(* Logix 5000 AddOnInstructionDefinition export EH_Liquitrend_QMW43_IOL; software revision 38.00 *)

TYPE EH_CommAOI_Data :
STRUCT
   Device_Comm_Error : BOOL;
   CommSuccess : BOOL;
   CommFailed : BOOL;
   CommTimeOut : BOOL;
   StateDone : BOOL;
   NewState : BOOL;
   OldState : SINT;
   PortSize : SINT;
   DevicePort : SINT;
   MaxState : SINT;
   State : SINT;
   VendorID : INT;
   DeviceID : DINT;
   CyclicData : INT[16];
   AcyclicData : DINT[8];
   ReplayIndex : INT;
   AOI_Diagnostic : DINT;
   ConnectionStatus : DINT;
   OutputData : INT[16];
END_STRUCT
END_TYPE

ADD_ON_INSTRUCTION EH_Liquitrend_QMW43_IOL   (* revision 1.0, vendor Endress+Hauser *)
// Liquitrend QMW43  Rev 1 IO-Link
VAR_IN_OUT
   DataToSend : INT[10]; {required}
   CommAOIBusy : DINT; {required}
   ActiveComPort : DINT; {required}
   DeviceAOISendRequest : DINT; {required}
   CommError : INT; {required}
   DeviceData : EH_CommAOI_Data; {required}
END_VAR
VAR_INPUT
   iExecuteRisingEdge : BOOL; {visible}
   iSetSimulation_Conductivity_Active : BOOL; {visible}
   iSetSimulation_Conductivity_Value : DINT; {visible}
   iSetSimulation_BuildUp_Active : BOOL; {visible}
   iSetSimulation_BuildUp_Value : INT; {visible}
END_VAR
VAR_OUTPUT
   qVendor_ID : DINT; {access Read Only, visible}
   qDevice_ID : DINT; {access Read Only, visible}
   qConductivity : REAL; {visible}
   qSimulationConductivityActive : BOOL; {visible}
   qBuildUp : REAL; {visible}
   qSimulationBuildUpActive : BOOL; {access Read Only, visible}
   qAOI_Diagnostic : DINT; {access Read Only, visible}
END_VAR
VAR_IN_OUT
   qActual_Diagnostics_String : STRING; {required}
END_VAR
VAR_OUTPUT
   qActual_Diagnostics_Code : DINT; {access Read Only, visible}
END_VAR
VAR_IN_OUT
   qLast_Diagnostics_String : STRING; {required}
END_VAR
VAR_OUTPUT
   qLast_Diagnostics_Code : DINT; {access Read Only, visible}
   qCommunicationBusy : DINT; {visible}
   qCommError : INT; {access Read Only, visible}
   qDeviceConnectionError : BOOL; {access Read Only, visible}
END_VAR
VAR
   Calc_DID : DINT; {access None}
   Calc_VID : DINT; {access None}
   Calc_Data : DINT; {access None}
   Conductivity_DINT : DINT; {access None}
   Calc_Conductivity : DINT; {access None}
   Calc_CondenStatus : DINT; {access None}
   CMD_Index : INT; {access None}
   CMD_Subindex : INT; {access None}
   CMD_ByteLength : INT; {access None}
   Calc_Connection_Status : DINT; {access None}
   Trigger : BOOL; {access None}
   CMD_Rd : BOOL; {access None}
   CMD_Wr : BOOL; {access None}
   Calc_Out : DINT; {access None}
   UnitSelection : REAL; {access None}
   InputByteLength : DINT;
   LocalChannel : BOOL; {access None}
   StateMin : DINT; {access None}
   UseDeviceUnit : BOOL; {access None}
   ActiveAOI : BOOL; {access None}
   firstTimeDone : BOOL; {access None}
   AOI_Prio : BOOL; {access None}
   BuidlUp_DINT : DINT;
   SimulationDINT : DINT; {access None}
   DeviceID1 : DINT; {access None}
   FALSE : BOOL; {access None}
   TRUE : BOOL := 1; {access None}
END_VAR

ROUTINE Logic   (* structured text *)
// PMP23 Communication via AL1323
   // ©Copyright (2024) All Rights Reserved
   // =======================================================================
   // Name:                EH_Liquitrend_QMW43_IOL
   // Version:             1.0
   // Datum:               11.2025
   // Library:             01.01.00
   // Engineering:         Studio5000 V38.00.00
   // Author:              EH
   // =======================================================================
   
   
   qAOI_Diagnostic := DeviceData.AOI_Diagnostic;
   qCommunicationBusy := CommAOIBusy;
   DeviceID1 := 1536;
   StateMin := 0;
   DeviceData.MaxState := 9;
   
   if DeviceData.DevicePort = 0 or DeviceData.DeviceID <> DeviceID1 or DeviceData.ConnectionStatus <> 1 then
   
   	qVendor_ID	:= 0;
   	qDevice_ID	:= 0;
   	qConductivity	:= 0;
   	qBuildUp	:=0;
   	qSimulationBuildUpActive	:= 0;
   	qSimulationConductivityActive	:= 0;
   	qActual_Diagnostics_Code	:= 0;
   	qLast_Diagnostics_Code	:= 0;
   	qLast_Diagnostics_String	:= '';
   
   	if DeviceData.DevicePort = 0 then
   
   		qActual_Diagnostics_String	:= 'Device Port is Zero';
   		DeviceData.AOI_Diagnostic.1 := TRUE;
   
   	elsif DeviceData.ConnectionStatus <> 1 then
   
   		qActual_Diagnostics_String	:= 'No Device connected';
   		qDeviceConnectionError := TRUE;
   
   	elsif DeviceData.DeviceID <> DeviceID1 then
   
   		qActual_Diagnostics_String	:= 'Wrong DeviceID';
   		DeviceData.AOI_Diagnostic.2 := TRUE;
   		qVendor_ID := DeviceData.VendorID;
   		qDevice_ID := DeviceData.DeviceID;
   
   	end_if;
   
   else
   
   	if qActual_Diagnostics_Code = 0 then
   
   		qActual_Diagnostics_String	:= '--------';
   
   	end_if;
   
   	if qLast_Diagnostics_Code = 0 then
   
   		qLast_Diagnostics_String	:= '--------';
   
   	end_if;
   
   	DeviceData.AOI_Diagnostic.1 := FALSE;
   	qDeviceConnectionError := FALSE;
   	DeviceData.AOI_Diagnostic.2  := FALSE;
   
   end_if;
   
   if NOT DeviceData.AOI_Diagnostic.0
   	and not qDeviceConnectionError
   	and not DeviceData.AOI_Diagnostic.2
   	and DeviceData.DevicePort > 0 or ActiveAOI and qDeviceConnectionError then
   
   	//*********************************
   	//Vendor ID
   	//*********************************
   
   	qVendor_ID := DeviceData.VendorID;
   
   	//*********************************
   	//Device ID
   	//*********************************
   
   	qDevice_ID := DeviceData.DeviceID;
   
   	//*********************************
   	//Process Data Conductivity
   	//*********************************
   
   		Calc_Conductivity := 0+((DeviceData.DevicePort-1)*InputByteLength);	// Value  95 + Protnumber x Datalength 32 Byte
   
   		Conductivity_DINT := DeviceData.CyclicData[Calc_Conductivity+1];
   		Conductivity_DINT.16 := DeviceData.CyclicData[Calc_Conductivity].0;
   		Conductivity_DINT.17 := DeviceData.CyclicData[Calc_Conductivity].1;
   		Conductivity_DINT.18 := DeviceData.CyclicData[Calc_Conductivity].2;
   		Conductivity_DINT.19 := DeviceData.CyclicData[Calc_Conductivity].3;
   		Conductivity_DINT.20 := DeviceData.CyclicData[Calc_Conductivity].4;
   		Conductivity_DINT.21 := DeviceData.CyclicData[Calc_Conductivity].5;
   		Conductivity_DINT.22 := DeviceData.CyclicData[Calc_Conductivity].6;
   		Conductivity_DINT.23 := DeviceData.CyclicData[Calc_Conductivity].7;
   		Conductivity_DINT.24 := DeviceData.CyclicData[Calc_Conductivity].7;
   		Conductivity_DINT.25 := DeviceData.CyclicData[Calc_Conductivity].7;
   		Conductivity_DINT.26 := DeviceData.CyclicData[Calc_Conductivity].7;
   		Conductivity_DINT.27 := DeviceData.CyclicData[Calc_Conductivity].7;
   		Conductivity_DINT.28 := DeviceData.CyclicData[Calc_Conductivity].7;
   		Conductivity_DINT.29 := DeviceData.CyclicData[Calc_Conductivity].7;
   		Conductivity_DINT.30 := DeviceData.CyclicData[Calc_Conductivity].7;
   		Conductivity_DINT.31 := DeviceData.CyclicData[Calc_Conductivity].7;
   		/*
   		Conductivity_DINT.0 := DeviceData.CyclicData[Calc_Conductivity+1].8;
   		Conductivity_DINT.1 := DeviceData.CyclicData[Calc_Conductivity+1].9;
   		Conductivity_DINT.2 := DeviceData.CyclicData[Calc_Conductivity+1].10;
   		Conductivity_DINT.3 := DeviceData.CyclicData[Calc_Conductivity+1].11;
   		Conductivity_DINT.4 := DeviceData.CyclicData[Calc_Conductivity+1].12;
   		Conductivity_DINT.5 := DeviceData.CyclicData[Calc_Conductivity+1].13;
   		Conductivity_DINT.6 := DeviceData.CyclicData[Calc_Conductivity+1].14;
   		Conductivity_DINT.7 := DeviceData.CyclicData[Calc_Conductivity+1].15;
   		Conductivity_DINT.8 := DeviceData.CyclicData[Calc_Conductivity+1].0;
   		Conductivity_DINT.9 := DeviceData.CyclicData[Calc_Conductivity+1].1;
   		Conductivity_DINT.10 := DeviceData.CyclicData[Calc_Conductivity+1].2;
   		Conductivity_DINT.11 := DeviceData.CyclicData[Calc_Conductivity+1].3;
   		Conductivity_DINT.12 := DeviceData.CyclicData[Calc_Conductivity+1].4;
   		Conductivity_DINT.13 := DeviceData.CyclicData[Calc_Conductivity+1].5;
   		Conductivity_DINT.14 := DeviceData.CyclicData[Calc_Conductivity+1].6;
   		Conductivity_DINT.15 := DeviceData.CyclicData[Calc_Conductivity+1].7;
   		Conductivity_DINT.16 := DeviceData.CyclicData[Calc_Conductivity].0;
   		Conductivity_DINT.17 := DeviceData.CyclicData[Calc_Conductivity].1;
   		Conductivity_DINT.18 := DeviceData.CyclicData[Calc_Conductivity].2;
   		Conductivity_DINT.19 := DeviceData.CyclicData[Calc_Conductivity].3;
   		Conductivity_DINT.20 := DeviceData.CyclicData[Calc_Conductivity].4;
   		Conductivity_DINT.21 := DeviceData.CyclicData[Calc_Conductivity].5;
   		Conductivity_DINT.22 := DeviceData.CyclicData[Calc_Conductivity].6;
   		Conductivity_DINT.23 := DeviceData.CyclicData[Calc_Conductivity].7;
   		Conductivity_DINT.24 := DeviceData.CyclicData[Calc_Conductivity].7;
   		Conductivity_DINT.25 := DeviceData.CyclicData[Calc_Conductivity].7;
   		Conductivity_DINT.26 := DeviceData.CyclicData[Calc_Conductivity].7;
   		Conductivity_DINT.27 := DeviceData.CyclicData[Calc_Conductivity].7;
   		Conductivity_DINT.28 := DeviceData.CyclicData[Calc_Conductivity].7;
   		Conductivity_DINT.29 := DeviceData.CyclicData[Calc_Conductivity].7;
   		Conductivity_DINT.30 := DeviceData.CyclicData[Calc_Conductivity].7;
   		Conductivity_DINT.31 := DeviceData.CyclicData[Calc_Conductivity].7;
   		*/
   
   		qConductivity := Conductivity_DINT;
   		qConductivity := qConductivity/10;
   
   	//*********************************
   	//Process Data BuildUp
   	//*********************************
   
   		BuidlUp_DINT.0 := DeviceData.CyclicData[Calc_Conductivity].8;
   		BuidlUp_DINT.1 := DeviceData.CyclicData[Calc_Conductivity].9;
   		BuidlUp_DINT.2 := DeviceData.CyclicData[Calc_Conductivity].10;
   		BuidlUp_DINT.3 := DeviceData.CyclicData[Calc_Conductivity].11;
   		BuidlUp_DINT.4 := DeviceData.CyclicData[Calc_Conductivity].12;
   		BuidlUp_DINT.5 := DeviceData.CyclicData[Calc_Conductivity].13;
   		BuidlUp_DINT.6 := DeviceData.CyclicData[Calc_Conductivity].14;
   		BuidlUp_DINT.7 := DeviceData.CyclicData[Calc_Conductivity].15;
   		BuidlUp_DINT.8 := DeviceData.CyclicData[Calc_Conductivity].15;
   		BuidlUp_DINT.9 := DeviceData.CyclicData[Calc_Conductivity].15;
   		BuidlUp_DINT.10 := DeviceData.CyclicData[Calc_Conductivity].15;
   		BuidlUp_DINT.11 := DeviceData.CyclicData[Calc_Conductivity].15;
   		BuidlUp_DINT.12 := DeviceData.CyclicData[Calc_Conductivity].15;
   		BuidlUp_DINT.13 := DeviceData.CyclicData[Calc_Conductivity].15;
   		BuidlUp_DINT.14 := DeviceData.CyclicData[Calc_Conductivity].15;
   		BuidlUp_DINT.15 := DeviceData.CyclicData[Calc_Conductivity].15;
   		BuidlUp_DINT.16 := DeviceData.CyclicData[Calc_Conductivity].15;
   		BuidlUp_DINT.17 := DeviceData.CyclicData[Calc_Conductivity].15;
   		BuidlUp_DINT.18 := DeviceData.CyclicData[Calc_Conductivity].15;
   		BuidlUp_DINT.19 := DeviceData.CyclicData[Calc_Conductivity].15;
   		BuidlUp_DINT.20 := DeviceData.CyclicData[Calc_Conductivity].15;
   		BuidlUp_DINT.21 := DeviceData.CyclicData[Calc_Conductivity].15;
   		BuidlUp_DINT.22 := DeviceData.CyclicData[Calc_Conductivity].15;
   		BuidlUp_DINT.23 := DeviceData.CyclicData[Calc_Conductivity].15;
   		BuidlUp_DINT.24 := DeviceData.CyclicData[Calc_Conductivity].15;
   		BuidlUp_DINT.25 := DeviceData.CyclicData[Calc_Conductivity].15;
   		BuidlUp_DINT.26 := DeviceData.CyclicData[Calc_Conductivity].15;
   		BuidlUp_DINT.27 := DeviceData.CyclicData[Calc_Conductivity].15;
   		BuidlUp_DINT.28 := DeviceData.CyclicData[Calc_Conductivity].15;
   		BuidlUp_DINT.29 := DeviceData.CyclicData[Calc_Conductivity].15;
   		BuidlUp_DINT.30 := DeviceData.CyclicData[Calc_Conductivity].15;
   		BuidlUp_DINT.31 := DeviceData.CyclicData[Calc_Conductivity].15;
   
   		qBuildUp := BuidlUp_DINT;
   		qBuildUp := qBuildUp/10;
   
   	//*********************************
   	// Checking for CommBlockBusy
   	//*********************************
   
   	if iExecuteRisingEdge and DeviceData.State = 0 then
   
   		DeviceAOISendRequest.[DeviceData.DevicePort] := 1;
   
   	end_if;
   
   	if ActiveComPort = DeviceData.DevicePort then
   
   		AOI_Prio :=1;
   	else
   
   		AOI_Prio := 0;
   	end_if;
   
   	if CommAOIBusy = 1 and iExecuteRisingEdge and DeviceData.State = 0 and AOI_Prio then
   
   		ActiveAOI := 1;
   
   	end_if;
   
   	qCommunicationBusy := CommAOIBusy;
   	qAOI_Diagnostic := DeviceData.AOI_Diagnostic;
   
   	if  ActiveAOI and qDeviceConnectionError then
   
   		DeviceData.State := DeviceData.MaxState;
   
   	end_if;
   
   	//*********************************
   	// State machine
   	//*********************************
   
   if ActiveAOI or DeviceData.State = DeviceData.MaxState then
   
   	case DeviceData.State of
   
   	    //*********************************
   	    0: // Idle
   	    //*********************************
   
   	    // Initializing
   	   		Trigger := 0;
   		    CMD_Index := 0;
   			CMD_Subindex := 0;
   	        CMD_Wr := 0;
   			CMD_Rd := 0;
   	        CMD_ByteLength := 0;
   
   			if DeviceData.DevicePort = ActiveComPort then // check if Device is Active to reset success
   					DeviceData.CommSuccess := 0;
   					DeviceData.CommTimeOut := 0;
   					DeviceData.NewState := 1;
   					DeviceData.StateDone := 0;
   			end_if;
   
   		    // Wait for trigger
   		    if iExecuteRisingEdge and ActiveComPort = DeviceData.DevicePort then
   
   				DeviceData.AOI_Diagnostic := 0;
   				DeviceData.State := DeviceData.State + 1;
   
   		    end_if;
   
   		//*********************************
   	    1: // Set Simulation Value Conductivity
   	    //*********************************
   
   	        CMD_Index := 86;
   	        CMD_Subindex := 0;
   	        CMD_Wr := 1;
   			CMD_Rd := 0;
   	        CMD_ByteLength := 4;
   			DataToSend[6]:= 0;
   			DataToSend[7]:= 0;
   
   			if iSetSimulation_Conductivity_Value <= 1100000 AND iSetSimulation_Conductivity_Value >= 0 then
   
   				COP(iSetSimulation_Conductivity_Value,SimulationDINT,1); // Copie the Bits from the Real in a DINT
   
   				DataToSend[6].0 :=  SimulationDINT.24;
   				DataToSend[6].1 :=  SimulationDINT.25;
   				DataToSend[6].2 :=  SimulationDINT.26;
   				DataToSend[6].3 :=  SimulationDINT.27;
   				DataToSend[6].4 :=  SimulationDINT.28;
   				DataToSend[6].5 :=  SimulationDINT.29;
   				DataToSend[6].6 :=  SimulationDINT.30;
   				DataToSend[6].7 :=  SimulationDINT.31;
   				DataToSend[6].8 :=  SimulationDINT.16;
   				DataToSend[6].9 :=  SimulationDINT.17;
   				DataToSend[6].10 := SimulationDINT.18;
   				DataToSend[6].11 := SimulationDINT.19;
   				DataToSend[6].12 := SimulationDINT.20;
   				DataToSend[6].13 := SimulationDINT.21;
   				DataToSend[6].14 := SimulationDINT.22;
   				DataToSend[6].15 := SimulationDINT.23;
   				DataToSend[7].0  := SimulationDINT.8;
   				DataToSend[7].1  := SimulationDINT.9;
   				DataToSend[7].2  := SimulationDINT.10;
   				DataToSend[7].3  := SimulationDINT.11;
   				DataToSend[7].4  := SimulationDINT.12;
   				DataToSend[7].5  := SimulationDINT.13;
   				DataToSend[7].6  := SimulationDINT.14;
   				DataToSend[7].7  := SimulationDINT.15;
   				DataToSend[7].8  := SimulationDINT.0;
   				DataToSend[7].9  := SimulationDINT.1;
   				DataToSend[7].10 := SimulationDINT.2;
   				DataToSend[7].11 := SimulationDINT.3;
   				DataToSend[7].12 := SimulationDINT.4;
   				DataToSend[7].13 := SimulationDINT.5;
   				DataToSend[7].14 := SimulationDINT.6;
   				DataToSend[7].15 := SimulationDINT.7;
   
   				Trigger := 1;
   
   				if DeviceData.NewState then
   
   					DeviceData.StateDone := 1;
   
   				end_if;
   
   				if  DeviceData.CommSuccess and DeviceData.ReplayIndex = CMD_Index then
   
   					Trigger := 0;
   					DeviceData.OldState := DeviceData.State;
   		    	    DeviceData.State := DeviceData.State + 1;
   					DeviceData.CommSuccess := 0;
   					DeviceData.AcyclicData[0] := 0;
   					DeviceData.NewState := 1;
   
   				 elsif DeviceData.CommTimeOut then
   
   					DeviceData.AOI_Diagnostic.[DeviceData.State+7] := 1;
   					DeviceData.OldState := DeviceData.State;
   		    	    DeviceData.State := DeviceData.State + 1;
   					DeviceData.CommTimeOut := 0;
   					DeviceData.AcyclicData[0] := 0;
   					DeviceData.NewState := 1;
   
   		    	end_if;
   
   			else
   
   				DeviceData.AOI_Diagnostic.[DeviceData.State+7] := 1;
   				DeviceData.OldState := DeviceData.State;
   		        DeviceData.State := DeviceData.State + 1;
   				DeviceData.CommTimeOut := 0;
   				DeviceData.AcyclicData[0] := 0;
   				DeviceData.NewState := 1;
   
   			end_if;
   
   		//*********************************
   		2: // Set Simulation Conductivity
   		//*********************************
   
   	        CMD_Index := 90;
   	        CMD_Subindex := 0;
   	        CMD_Wr := 1;
   			CMD_Rd := 0;
   	        CMD_ByteLength := 1;
   			DataToSend[6]:= 0;
   			DataToSend[7]:= 0;
   
   			DataToSend[6].0 := iSetSimulation_Conductivity_Active;
   			Trigger := 1;
   
   			if DeviceData.NewState then
   
   				DeviceData.StateDone := 1;
   
   			end_if;
   
   			if  DeviceData.CommSuccess and DeviceData.ReplayIndex = CMD_Index then
   
   					Trigger := 0;
   					DeviceData.OldState := DeviceData.State;
   			        DeviceData.State := DeviceData.State + 1;
   					DeviceData.CommSuccess := 0;
   					DeviceData.AcyclicData[0] := 0;
   					DeviceData.NewState := 1;
   
   			 elsif DeviceData.CommTimeOut then
   
   					DeviceData.AOI_Diagnostic.[DeviceData.State+7] := 1;
   					DeviceData.OldState := DeviceData.State;
   			        DeviceData.State := DeviceData.State + 1;
   					DeviceData.CommTimeOut := 0;
   					DeviceData.AcyclicData[0] := 0;
   					DeviceData.NewState := 1;
   
   			   end_if;
   
   		//*********************************
   	    3: // Set Simulation Value BuildUP
   	    //*********************************
   
   	        CMD_Index := 85;
   	        CMD_Subindex := 0;
   	        CMD_Wr := 1;
   			CMD_Rd := 0;
   	        CMD_ByteLength := 2;
   			DataToSend[6]:= 0;
   			DataToSend[7]:= 0;
   
   			if iSetSimulation_BuildUp_Value <= 100 or iSetSimulation_BuildUp_Value >= 0 then
   
   				COP(iSetSimulation_BuildUp_Value,SimulationDINT,1); // Copie the Bits from the Real in a DINT
   
   				DataToSend[6].0  := SimulationDINT.8;
   				DataToSend[6].1  := SimulationDINT.9;
   				DataToSend[6].2  := SimulationDINT.10;
   				DataToSend[6].3  := SimulationDINT.11;
   				DataToSend[6].4  := SimulationDINT.12;
   				DataToSend[6].5  := SimulationDINT.13;
   				DataToSend[6].6  := SimulationDINT.14;
   				DataToSend[6].7  := SimulationDINT.15;
   				DataToSend[6].8  := SimulationDINT.0;
   				DataToSend[6].9  := SimulationDINT.1;
   				DataToSend[6].10 := SimulationDINT.2;
   				DataToSend[6].11 := SimulationDINT.3;
   				DataToSend[6].12 := SimulationDINT.4;
   				DataToSend[6].13 := SimulationDINT.5;
   				DataToSend[6].14 := SimulationDINT.6;
   				DataToSend[6].15 := SimulationDINT.7;
   
   				Trigger := 1;
   
   				if DeviceData.NewState then
   
   					DeviceData.StateDone := 1;
   
   				end_if;
   
   				if  DeviceData.CommSuccess and DeviceData.ReplayIndex = CMD_Index then
   
   					Trigger := 0;
   					DeviceData.OldState := DeviceData.State;
   			        DeviceData.State := DeviceData.State + 1;
   					DeviceData.CommSuccess := 0;
   					DeviceData.AcyclicData[0] := 0;
   					DeviceData.NewState := 1;
   
   				 elsif DeviceData.CommTimeOut then
   
   					DeviceData.AOI_Diagnostic.[DeviceData.State+7] := 1;
   					DeviceData.OldState := DeviceData.State;
   			        DeviceData.State := DeviceData.State + 1;
   					DeviceData.CommTimeOut := 0;
   					DeviceData.AcyclicData[0] := 0;
   					DeviceData.NewState := 1;
   
   			    end_if;
   
   			else
   
   				DeviceData.AOI_Diagnostic.[DeviceData.State+7] := 1;
   				DeviceData.OldState := DeviceData.State;
   		        DeviceData.State := DeviceData.State + 1;
   				DeviceData.CommTimeOut := 0;
   				DeviceData.AcyclicData[0] := 0;
   				DeviceData.NewState := 1;
   
   			end_if;
   
   
   		//*********************************
   		4: // Set Simulation BuildUP
   		//*********************************
   
   	        CMD_Index := 66;
   	        CMD_Subindex := 0;
   	        CMD_Wr := 1;
   			CMD_Rd := 0;
   	        CMD_ByteLength := 1;
   			DataToSend[6]:= 0;
   			DataToSend[7]:= 0;
   
   			DataToSend[6].0 := iSetSimulation_Conductivity_Active;
   			Trigger := 1;
   
   			if DeviceData.NewState then
   
   				DeviceData.StateDone := 1;
   
   			end_if;
   
   			if  DeviceData.CommSuccess and DeviceData.ReplayIndex = CMD_Index then
   
   					Trigger := 0;
   					DeviceData.OldState := DeviceData.State;
   			        DeviceData.State := DeviceData.State + 1;
   					DeviceData.CommSuccess := 0;
   					DeviceData.AcyclicData[0] := 0;
   					DeviceData.NewState := 1;
   
   			 elsif DeviceData.CommTimeOut then
   
   					DeviceData.AOI_Diagnostic.[DeviceData.State+7] := 1;
   					DeviceData.OldState := DeviceData.State;
   			        DeviceData.State := DeviceData.State + 1;
   					DeviceData.CommTimeOut := 0;
   					DeviceData.AcyclicData[0] := 0;
   					DeviceData.NewState := 1;
   
   			   end_if;
   
   		//*********************************
   	    5: // Read Simulation Conductivity Active
   	    //*********************************
   
   			CMD_Index := 90;
   	        CMD_Subindex := 0;
   	        CMD_Wr := 0;
   			CMD_Rd := 1;
   	        CMD_ByteLength := 1;
   			DataToSend[6]:= 0;
   			DataToSend[7]:= 0;
   			Trigger := 1;
   
   			if DeviceData.NewState then
   
   				DeviceData.StateDone := 1;
   
   			end_if;
   
   			if  DeviceData.CommSuccess and DeviceData.ReplayIndex = CMD_Index then
   
   				qSimulationConductivityActive := DeviceData.AcyclicData[0].0;
   
   				Trigger := 0;
   				DeviceData.OldState := DeviceData.State;
   		        DeviceData.State := DeviceData.State + 1;
   				DeviceData.CommSuccess := 0;
   				DeviceData.AcyclicData[0] := 0;
   				DeviceData.NewState := 1;
   
   			 elsif DeviceData.CommTimeOut then
   
   				DeviceData.AOI_Diagnostic.[DeviceData.State+7] := 1;
   				DeviceData.OldState := DeviceData.State;
   		        DeviceData.State := DeviceData.State + 1;
   				DeviceData.CommTimeOut := 0;
   				DeviceData.AcyclicData[0] := 0;
   				DeviceData.NewState := 1;
   
   		    end_if;
   
   		//*********************************
   	    6: // Read Simulation BuildUp Active
   	    //*********************************
   
   			CMD_Index := 66;
   	        CMD_Subindex := 0;
   	        CMD_Wr := 0;
   			CMD_Rd := 1;
   	        CMD_ByteLength := 1;
   			DataToSend[6]:= 0;
   			DataToSend[7]:= 0;
   			Trigger := 1;
   
   			if DeviceData.NewState then
   
   				DeviceData.StateDone := 1;
   
   			end_if;
   
   			if  DeviceData.CommSuccess and DeviceData.ReplayIndex = CMD_Index then
   
   				qSimulationBuildUpActive := DeviceData.AcyclicData[0].0;
   
   				Trigger := 0;
   				DeviceData.OldState := DeviceData.State;
   		        DeviceData.State := DeviceData.State + 1;
   				DeviceData.CommSuccess := 0;
   				DeviceData.AcyclicData[0] := 0;
   				DeviceData.NewState := 1;
   
   			 elsif DeviceData.CommTimeOut then
   
   				DeviceData.AOI_Diagnostic.[DeviceData.State+7] := 1;
   				DeviceData.OldState := DeviceData.State;
   		        DeviceData.State := DeviceData.State + 1;
   				DeviceData.CommTimeOut := 0;
   				DeviceData.AcyclicData[0] := 0;
   				DeviceData.NewState := 1;
   
   		    end_if;
   
   		//*********************************
   	    7: // Actual Diagnostic
   	    //*********************************
   
   	        CMD_Index := 260;
   	        CMD_Subindex := 0;
   	        CMD_Wr := 0;
   			CMD_Rd := 1;
   			CMD_ByteLength := 2;
   
   			Trigger := 1;
   
   			if DeviceData.NewState then
   
   				DeviceData.StateDone := 1;
   
   			end_if;
   
   			if  DeviceData.CommSuccess and DeviceData.ReplayIndex = CMD_Index then
   
   				qActual_Diagnostics_Code	:= DeviceData.AcyclicData[0];
   
   				case qActual_Diagnostics_Code of
   
   					16#2D20_2D20:
   		    	       qActual_Diagnostics_String := 'SYSTEM OK';
   					16#0000_0001:
   						qActual_Diagnostics_String := 'no communication';
   					16#4632_3730:
   					    qActual_Diagnostics_String := 'F270 - Defect in electronic / sensor';
   					16#5338_3034:
   					    qActual_Diagnostics_String := 'S804 - Load current > 200mA per output';
   					16#4334_3835:
   					    qActual_Diagnostics_String := 'C485 - Simulation active';
   					16#4331_3832:
   					    qActual_Diagnostics_String := 'C182 - Invalid calibration';
   					16#4331_3033:
   					    qActual_Diagnostics_String := 'C103 - Sensor check failed';
   					16#5338_3235:
   					    qActual_Diagnostics_String := 'S825 - Ambient temperature out of specification';
   				else
   						qActual_Diagnostics_String := 'Error Code unknown';
   
   		 		end_case;
   
   				Trigger := 0;
   				DeviceData.OldState := DeviceData.State;
   		        DeviceData.State := DeviceData.State + 1;
   				DeviceData.CommSuccess := 0;
   				DeviceData.AcyclicData[0] := 0;
   				DeviceData.NewState := 1;
   
   			elsif DeviceData.CommTimeOut then
   
   				DeviceData.AOI_Diagnostic.[DeviceData.State+7] := 1;
   				Trigger := 0;
   				DeviceData.OldState := DeviceData.State;
   		        DeviceData.State := DeviceData.State + 1;
   				DeviceData.CommTimeOut := 0;
   				DeviceData.AcyclicData[0] := 0;
   				DeviceData.NewState := 1;
   
   		    end_if;
   
   		//*********************************
   	   	8: // Last Diagnostic
   	    //*********************************
   
   	        CMD_Index := 261;
   			CMD_Subindex := 0;
   	        CMD_Wr := 0;
   			CMD_Rd := 1;
   			CMD_ByteLength := 2;
   	        Trigger := 1;
   
   			if DeviceData.NewState then
   
   				DeviceData.StateDone := 1;
   
   			end_if;
   
   			if  DeviceData.CommSuccess and DeviceData.ReplayIndex = CMD_Index then
   
   				qLast_Diagnostics_Code	:= DeviceData.AcyclicData[0];
   
   				case qLast_Diagnostics_Code of
   
   					16#2D20_2D20:
   		    	      qLast_Diagnostics_String := 'SYSTEM OK';
   					16#0000_0001:
   						qLast_Diagnostics_String := 'no communication';
   					16#4632_3730:
   					    qLast_Diagnostics_String := 'F270 - Defect in electronic / sensor';
   					16#5338_3034:
   					    qLast_Diagnostics_String := 'S804 - Load current > 200mA per output';
   					16#4334_3835:
   					    qLast_Diagnostics_String := 'C485 - Simulation active';
   					16#4331_3832:
   					    qLast_Diagnostics_String := 'C182 - Invalid calibration';
   					16#4331_3033:
   					    qLast_Diagnostics_String := 'C103 - Sensor check failed';
   					16#5338_3235:
   					    qLast_Diagnostics_String := 'S825 - Ambient temperature out of specification';
   				else
   						qLast_Diagnostics_String := 'Error Code unknown';
   
   		 		end_case;
   
   				Trigger := 0;
   				DeviceData.OldState := DeviceData.State;
   		        DeviceData.State := DeviceData.State + 1;
   				DeviceData.CommSuccess := 0;
   				DeviceData.AcyclicData[0] := 0;
   				DeviceData.NewState := 1;
   
   			elsif DeviceData.CommTimeOut then
   
   				DeviceData.AOI_Diagnostic.[DeviceData.State+7] := 1;
   				Trigger := 0;
   				DeviceData.OldState := DeviceData.State;
   		        DeviceData.State := DeviceData.State + 1;
   				DeviceData.CommTimeOut := 0;
   				DeviceData.AcyclicData[0] := 0;
   				DeviceData.NewState := 1;
   
   		    end_if;
   
   		//*********************************
   	    9: // Trigger guard
   	    //*********************************
   
   			if not firstTimeDone then
   
   				CommAOIBusy := 0;
   				firstTimeDone := 1;
   				DeviceAOISendRequest.[DeviceData.DevicePort] := 0;
   				ActiveComPort := 0;
   				ActiveAOI := 0;
   				DataToSend[0] := 0;
   				DataToSend[1] := 0;
   				DataToSend[2] := 0;
   				DataToSend[3] := 0;
   				DataToSend[4] := 0;
   				DataToSend[5] := 0;
   				DataToSend[6] := 0;
   				DataToSend[7] := 0;
   				DataToSend[8] := 0;
   				DataToSend[9] := 0;
   				DeviceData.StateDone := 0;
   
   			end_if;
   
   			if DeviceData.State = DeviceData.MaxState AND NOT iExecuteRisingEdge then
   
   				DeviceData.State := 0;
   				DeviceData.OldState := DeviceData.State;
   				firstTimeDone := 0;
   
   			end_if;
   
   		end_case;
   
   end_if;
   
   	//*************************
   	// Write Commands to the Master and the Device
   	//*************************
   	if DeviceData.State > StateMin and DeviceData.State < DeviceData.MaxState then
   
   		DataToSend[2] :=  DeviceData.DevicePort;
   		DataToSend[3] := CMD_Index;
   		DataToSend[4] := CMD_Subindex;
   		DataToSend[5].0 := CMD_Rd;
   		DataToSend[5].1 := CMD_Wr;
   		DataToSend[5].8 := CMD_ByteLength.0;
   		DataToSend[5].9 := CMD_ByteLength.1;
   		DataToSend[5].10 := CMD_ByteLength.2;
   		DataToSend[5].11 := CMD_ByteLength.3;
   		DataToSend[5].12 := CMD_ByteLength.4;
   		DataToSend[5].13 := CMD_ByteLength.5;
   		DataToSend[5].14 := CMD_ByteLength.6;
   		DataToSend[5].15 := CMD_ByteLength.7;
   
   		DataToSend[5].7 := Trigger;
   
   		qCommError	:= CommError;
   
   	end_if;
   
   end_if;
END_ROUTINE
END_ADD_ON_INSTRUCTION
